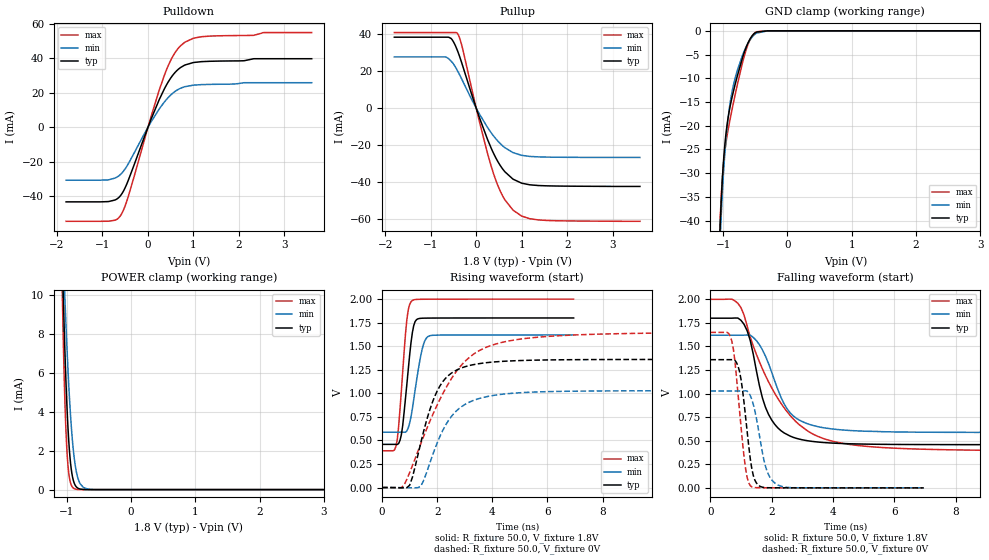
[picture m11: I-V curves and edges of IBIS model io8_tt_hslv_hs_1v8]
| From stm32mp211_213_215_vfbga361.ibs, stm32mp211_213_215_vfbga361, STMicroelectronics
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[Model]   io8_tt_hslv_hs_1v8
Model_type I/O
Polarity   Non-Inverting
Enable   Active-Low
| CAP_THRESHOLD on pad IOTT is "UDTCAPC" :
| Rising=30.0% of vddiov33m   Falling=70.0% of vddiov33m
| C_comp min and max val. don't necessarily correlate with the min and max pvt
| but are the smallest and greatest pad capacitance found.
| var   typ   min   max
C_comp   1.26690pF  1.09321pF  1.36430pF
|C_comp_pullup   869.30000fF  531.82000fF  521.19000fF
|C_comp_pulldown   397.59601fF  561.39043fF  843.10518fF
Vinl = 810.0mV
Vinh = 1.0V
Vmeas = 900.0mV   | Reference voltage for timing measurements
Cref  = 50.0pF   | Timing specification test load capacitance value
Rref  = 1.0MOhm   | Timing specification test load resistance value
Vref  = 990.0mV   | Timing specification test load voltage
[Model Spec]
| TIME_THRESHOLD on pin ZIV08M is "CMOS" :
| Rising=50.0% of vddv08m   Falling=50.0% of vddv08m
Vinl 675.70000mV 623.70000mV 735.70000mV
Vinh 1.12730V 1.01130V 1.24930V
| variable   typ   min   max
[Temperature Range] 25.0 125.0 -40.0
| variable   typ   min   max
[Voltage Range] 1.8V 1.62V 2.0V
| variable   typ   min   max
[POWER Clamp Reference] 1.8V 1.62V 2.0V
| variable   typ   min   max
[GND Clamp Reference] 0V 0V 0V
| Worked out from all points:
|   slope of the pulldown table from 0 to 0.27 V, typ, clamps not added: 15.6 ohm
|   slope of the pullup table from 0 to 0.27 V, typ, clamps not added: 14.9 ohm
|   GND clamp passes 1 mA (typ) near -0.55 V on its own axis
|   POWER clamp passes 1 mA (typ) near -0.93 V on its own axis
|   rising waveform, R_fixture 50.0, V_fixture 1.8V: 20-80 % time 274ps typ, 339ps min, 247ps max; typ from 0.458 V to 1.8 V
|   falling waveform, R_fixture 50.0, V_fixture 1.8V: 20-80 % time 666ps typ, 835ps min, 1.53ns max; typ from 1.8 V to 0.458 V
|   rising waveform, R_fixture 50.0, V_fixture 0V: 20-80 % time 880ps typ, 1.06ns min, 1.71ns max; typ from 0 V to 1.36 V
|   falling waveform, R_fixture 50.0, V_fixture 0V: 20-80 % time 292ps typ, 372ps min, 291ps max; typ from 1.36 V to 0 V
[POWER Clamp]
-1.8V     152.1mA    105.6mA    221.1mA
-1.07V    12.07mA    13.62mA    10.38mA
-1.05V    9.569mA    11.75mA    7.249mA
-1.03V    7.339mA    9.993mA    4.743mA
-1.01V    5.42mA     8.357mA    2.898mA
-990mV    3.841mA    6.859mA    1.662mA
-970mV    2.609mA    5.513mA    906.5uA
-940mV    1.358mA    3.806mA    344.1uA
-880mV    308.3uA    1.548mA    45.55uA
-790mV    28.47uA    298.6uA    2.144uA
-610mV    219.5nA    7.365uA    27.8nA
3.6V      0A         0A         0A
[GND Clamp]
-1.8V     -1.222A    -1.193A    -1.238A
-1.05V    -42.33mA   -45.55mA   -41.2mA
-1.04V    -38.89mA   -42.1mA    -37.88mA
-1.03V    -35.83mA   -38.98mA   -35.06mA
-1.01V    -30.7mA    -33.54mA   -30.61mA
-970mV    -23.47mA   -25.17mA   -24.97mA
-920mV    -18.06mA   -18.06mA   -20.63mA
-870mV    -14.51mA   -13.44mA   -17.13mA
-780mV    -9.532mA   -8.354mA   -11.38mA
-650mV    -3.743mA   -3.581mA   -4.327mA
-490mV    -324.1uA   -556uA     -259.6uA
3.6V      67.14nA    3.404uA    33.72nA
| variable   typ   min   max
[Pullup Reference] 1.8V 1.62V 2.0V
| variable   typ   min   max
[Pulldown Reference] 0V 0V 0V
[Pullup]
-1.8V     38.22mA    27.62mA    40.72mA
-610mV    38.2mA     26.68mA    40.72mA
-520mV    36.51mA    24.52mA    40.72mA
-410mV    30.85mA    20.07mA    40.15mA
-310mV    23.77mA    15.24mA    33.09mA
70mV      -5.022mA   -3.131mA   -7.212mA
350mV     -22.69mA   -13.97mA   -32.92mA
570mV     -32.38mA   -20.06mA   -46.75mA
810mV     -38.27mA   -23.98mA   -54.98mA
1V        -40.44mA   -25.43mA   -58.16mA
1.37V     -41.7mA    -26.27mA   -60.24mA
3.6V      -42.18mA   -26.58mA   -60.97mA
[Pulldown]
-1.8V     -43.21mA   -30.64mA   -54.48mA
-870mV    -43.06mA   -30.5mA    -54.44mA
-700mV    -41.81mA   -29.1mA    -53.55mA
-600mV    -39.48mA   -27.21mA   -51.03mA
-440mV    -31.2mA    -21.48mA   -40.66mA
70mV      4.786mA    3.206mA    6.392mA
360mV     22.22mA    14.64mA    30.08mA
580mV     31.3mA     20.48mA    42.61mA
810mV     36.07mA    23.54mA    49.29mA
1.18V     38.05mA    24.73mA    52.5mA
2.54V     39.74mA    25.83mA    54.9mA
3.6V      39.74mA    25.83mA    54.9mA
[Ramp]
dV/dt_r 815.91813mV/877.91674ps 616.4941mV/1.05884ns 989.55702mV/1.7123ns
dV/dt_f 805.07322mV/661.55151ps 619.1849mV/832.54737ps 965.62698mV/1.52645ns
R_load = 50.0
| Removed startup time: 0s 0s 0s  .
| Removed end time: 6.95ns.
[Rising Waveform]
R_fixture   = 50.0
V_fixture   = 1.8V
V_fixture_min = 1.62V
V_fixture_max = 2.0V
0s        458.2mV    588mV      390.6mV
450ps     458.2mV    588mV      399mV
550ps     456.9mV    588mV      506mV
700ps     560.7mV    588mV      1.024V
900ps     1.097V     601.7mV    1.783V
1.1ns     1.645V     837.3mV    1.986V
1.2ns     1.762V     1.037V     1.995V
1.45ns    1.797V     1.462V     1.999V
1.7ns     1.799V     1.608V     1.999V
6.95ns    1.8V       1.62V      2V
| Removed startup time: 0s 0s 0s  .
| Removed end time: 199.9ns.
[Falling Waveform]
R_fixture   = 50.0
V_fixture   = 1.8V
V_fixture_min = 1.62V
V_fixture_max = 2.0V
0s        1.8V       1.62V      2V
700ps     1.8V       1.62V      2.002V
1.1ns     1.735V     1.62V      1.833V
1.3ns     1.566V     1.62V      1.601V
1.8ns     852.7mV    1.395V     1.189V
2.4ns     583.6mV    893.6mV    851.6mV
2.9ns     517.1mV    718.8mV    669.5mV
3.8ns     478.6mV    632.3mV    511.2mV
7ns       459.3mV    590.4mV    409.4mV
199.9ns   458.2mV    588mV      390.6mV
| Removed startup time: 0s 0s 0s  .
| Removed end time: 199.9ns.
[Rising Waveform]
R_fixture   = 50.0
V_fixture   = 0V
V_fixture_min = 0V
V_fixture_max = 0V
0s        126.9nV    1.961uV    185.2nV
700ps     -2.867mV   -6.099uV   -1.827mV
1ns       24.28mV    -1.989mV   158.5mV
1.4ns     468.8mV    12.81mV    460.9mV
1.9ns     960.4mV    397.9mV    813.6mV
2.6ns     1.23V      784.3mV    1.193V
3.3ns     1.304V     923.1mV    1.412V
4.1ns     1.334V     980.4mV    1.521V
7.8ns     1.358V     1.025V     1.628V
199.9ns   1.36V      1.027V     1.649V
| Removed startup time: 0s 0s 0s  .
| Removed end time: 6.95ns.
[Falling Waveform]
R_fixture   = 50.0
V_fixture   = 0V
V_fixture_min = 0V
V_fixture_max = 0V
0s        1.36V      1.027V     1.649V
700ps     1.36V      1.028V     1.558V
800ps     1.354V     1.027V     1.348V
1ns       1.153V     1.027V     651.7mV
1.2ns     600.5mV    1.026V     110.5mV
1.35ns    208mV      940.9mV    10.8mV
1.5ns     52.77mV    742.2mV    2.241mV
1.8ns     2.563mV    226.6mV    887.2uV
2.2ns     654.5uV    31.1mV     465uV
6.95ns    14.41uV    29.73uV    37.39uV
